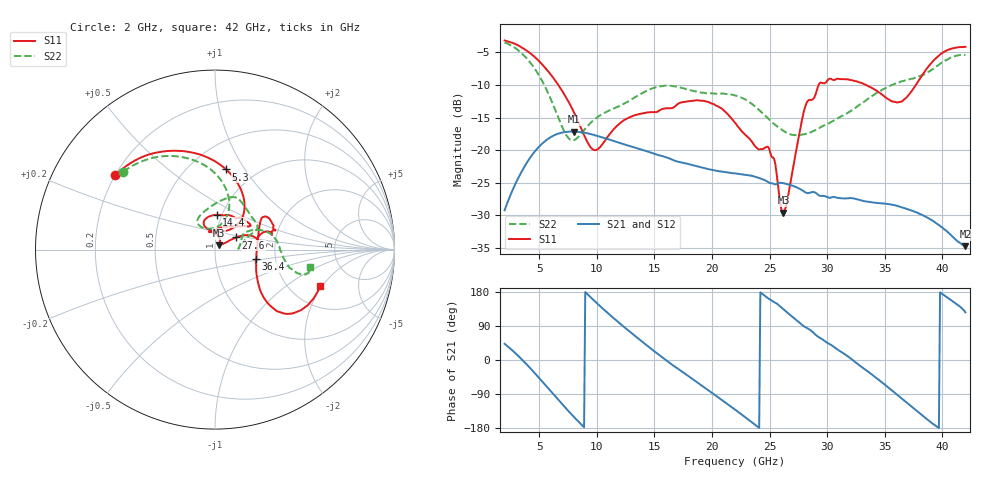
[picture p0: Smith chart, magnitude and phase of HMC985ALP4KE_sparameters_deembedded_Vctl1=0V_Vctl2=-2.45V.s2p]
!s2p File: Measurements: S11, S21, S12, S22
# GHz S dB R 50.0
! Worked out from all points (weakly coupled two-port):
!   401 points, 2 GHz to 42 GHz, reference 50 ohm
!   highest |S21| = -17.15 dB at 8 GHz (marker M1); lowest = -34.7 dB at 42 GHz (marker M2)
!   lowest |S11| = -29.6 dB at 26.2 GHz (marker M3), VSWR 1.07, Z = 52.3 + j2.51 ohm
!   |S11| at or under -10 dB: 6.662 GHz to 29.26 GHz (22.6 GHz wide, 126 % of centre); 33.37 GHz to 37.7 GHz (4.325 GHz wide, 12.2 % of centre)
!   |S22| runs from -18.5 to -3.5 dB; largest |S21 - S12| = 0.00055
!   S11 on the Smith chart (normalised r, x): 2 GHz: 0.20, +0.32; 5.3 GHz: 0.74, +0.83; 14.4 GHz: 0.94, +0.38; 27.6 GHz: 1.25, +0.17; 36.4 GHz: 1.58, -0.18; 42 GHz: 2.91, -1.91
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2  -3.17 143.3  -29.22 42.7  -29.21 42.7  -3.48 139.6
3.5  -4.26 116.4  -23.21 1.4  -23.23 1.3  -5.17 110.3
5.3  -6.92 82.1  -18.93 -58.0  -18.95 -58.1  -9.52 78.8
8  -14.12 48.2  -17.15 -149.6  -17.13 -149.6  -18.47 101.6
8.7  -16.89 52.5  -17.25 -171.5  -17.24 -171.5  -17.36 117.4
9.9  -19.99 86.8  -17.73 153.0  -17.73 153.0  -15.13 123.3
12.2  -15.61 112.1  -19.00 91.5  -18.99 91.5  -13.02 104.1
14.4  -14.21 87.1  -20.19 37.2  -20.17 37.3  -10.84 79.3
15.4  -13.95 73.5  -20.78 13.8  -20.80 13.8  -10.23 71.9
19.3  -12.43 34.0  -22.73 -71.5  -22.75 -71.5  -11.18 43.1
22  -15.77 52.3  -23.57 -130.8  -23.59 -130.9  -11.60 26.3
25  -19.96 98.9  -25.03 160.4  -24.99 160.4  -15.36 17.1
26.2  -29.57 46.1  -25.06 134.0  -25.09 133.9  -17.03 7.6
27.6  -17.34 29.8  -25.91 97.9  -25.92 97.8  -17.64 2.6
28.1  -13.29 20.9  -26.45 86.7  -26.49 86.7  -17.52 4.3
28.7  -12.26 13.0  -26.42 75.0  -26.43 75.0  -17.14 8.3
31  -9.06 23.3  -27.34 25.8  -27.32 25.7  -15.02 28.1
33.3  -9.93 34.2  -27.84 -25.0  -27.84 -25.0  -12.46 26.9
35.4  -12.27 12.0  -28.29 -74.8  -28.27 -74.9  -10.19 18.1
36.4  -12.58 -13.1  -28.71 -99.9  -28.74 -100.0  -9.46 12.3
39.5  -5.82 -43.4  -31.25 -175.1  -31.18 -175.5  -7.12 -14.2
42  -4.15 -19.0  -34.72 125.6  -34.71 125.7  -5.37 -10.1
